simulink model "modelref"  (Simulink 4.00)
settings: Solver=ode45  StartTime=0.0  StopTime=1000.0  RelTol=1e-3
libraries: simulink3 x3

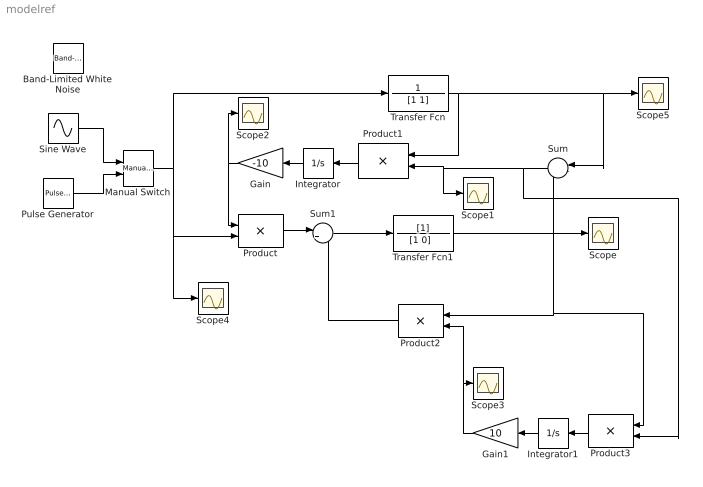
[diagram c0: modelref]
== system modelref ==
  Band-Limited White Noise : simulink3/Sources/Band-Limited White Noise  Cov=[0.1]  Ts=10  seed=[23341]
  Gain : Gain  Orientation=left  Gain=-10  Multiplication=Element-wise(K.*u)  SaturateOnIntegerOverflow=on
  Gain1 : Gain  Orientation=left  Gain=10  Multiplication=Element-wise(K.*u)  SaturateOnIntegerOverflow=on
  Integrator : Integrator  Orientation=left  ExternalReset=none  InitialConditionSource=internal  InitialCondition=0  LimitOutput=off  UpperSaturationLimit=inf  LowerSaturationLimit=-inf  ShowSaturationPort=off  ShowStatePort=off  AbsoluteTolerance=auto
  Integrator1 : Integrator  Orientation=left  ExternalReset=none  InitialConditionSource=internal  InitialCondition=0  LimitOutput=off  UpperSaturationLimit=inf  LowerSaturationLimit=-inf  ShowSaturationPort=off  ShowStatePort=off  AbsoluteTolerance=auto
  Manual Switch : simulink3/Nonlinear/Manual Switch  sw=0  action=0
  Product : Product  Inputs=2  Multiplication=Element-wise(.*)  SaturateOnIntegerOverflow=on
  Product1 : Product  Orientation=left  Inputs=2  Multiplication=Element-wise(.*)  SaturateOnIntegerOverflow=on
  Product2 : Product  Orientation=left  Inputs=2  Multiplication=Element-wise(.*)  SaturateOnIntegerOverflow=on
  Product3 : Product  Orientation=left  Inputs=2  Multiplication=Element-wise(.*)  SaturateOnIntegerOverflow=on
  Pulse Generator : simulink3/Sources/Pulse Generator  period=10  duty=50  amplitude=1  start=0
  Scope{,1..5} (6 alike) : Scope
  Sine Wave : Sin  Amplitude=1  Frequency=.1  Phase=0  SampleTime=0
  Sum : Sum  Orientation=left  Inputs=|-+  SaturateOnIntegerOverflow=on
  Sum1 : Sum  Inputs=|+-  SaturateOnIntegerOverflow=on
  Transfer Fcn : TransferFcn  Numerator=1  Denominator=[1 1]  Realization=auto  AbsoluteTolerance=auto
  Transfer Fcn1 : TransferFcn  Numerator=[1]  Denominator=[1 0]  Realization=auto  AbsoluteTolerance=auto
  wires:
  Transfer Fcn1/1 -> Scope/1, Sum/2, Product2/1, Product3/1
  Transfer Fcn/1 -> Product1/1, Sum/1, Scope5/1
  Integrator/1 -> Gain/1
  Gain/1 -> Product/1, Scope2/1
  Product1/1 -> Integrator/1
  Sum/1 -> Product1/2, Scope1/1, Product3/2
  Pulse Generator/1 -> Manual Switch/2
  Manual Switch/1 -> Transfer Fcn/1, Product/2, Scope4/1
  Product/1 -> Sum1/1
  Sum1/1 -> Transfer Fcn1/1
  Product2/1 -> Sum1/2
  Integrator1/1 -> Gain1/1
  Gain1/1 -> Scope3/1, Product2/2
  Product3/1 -> Integrator1/1
  Sine Wave/1 -> Manual Switch/1
